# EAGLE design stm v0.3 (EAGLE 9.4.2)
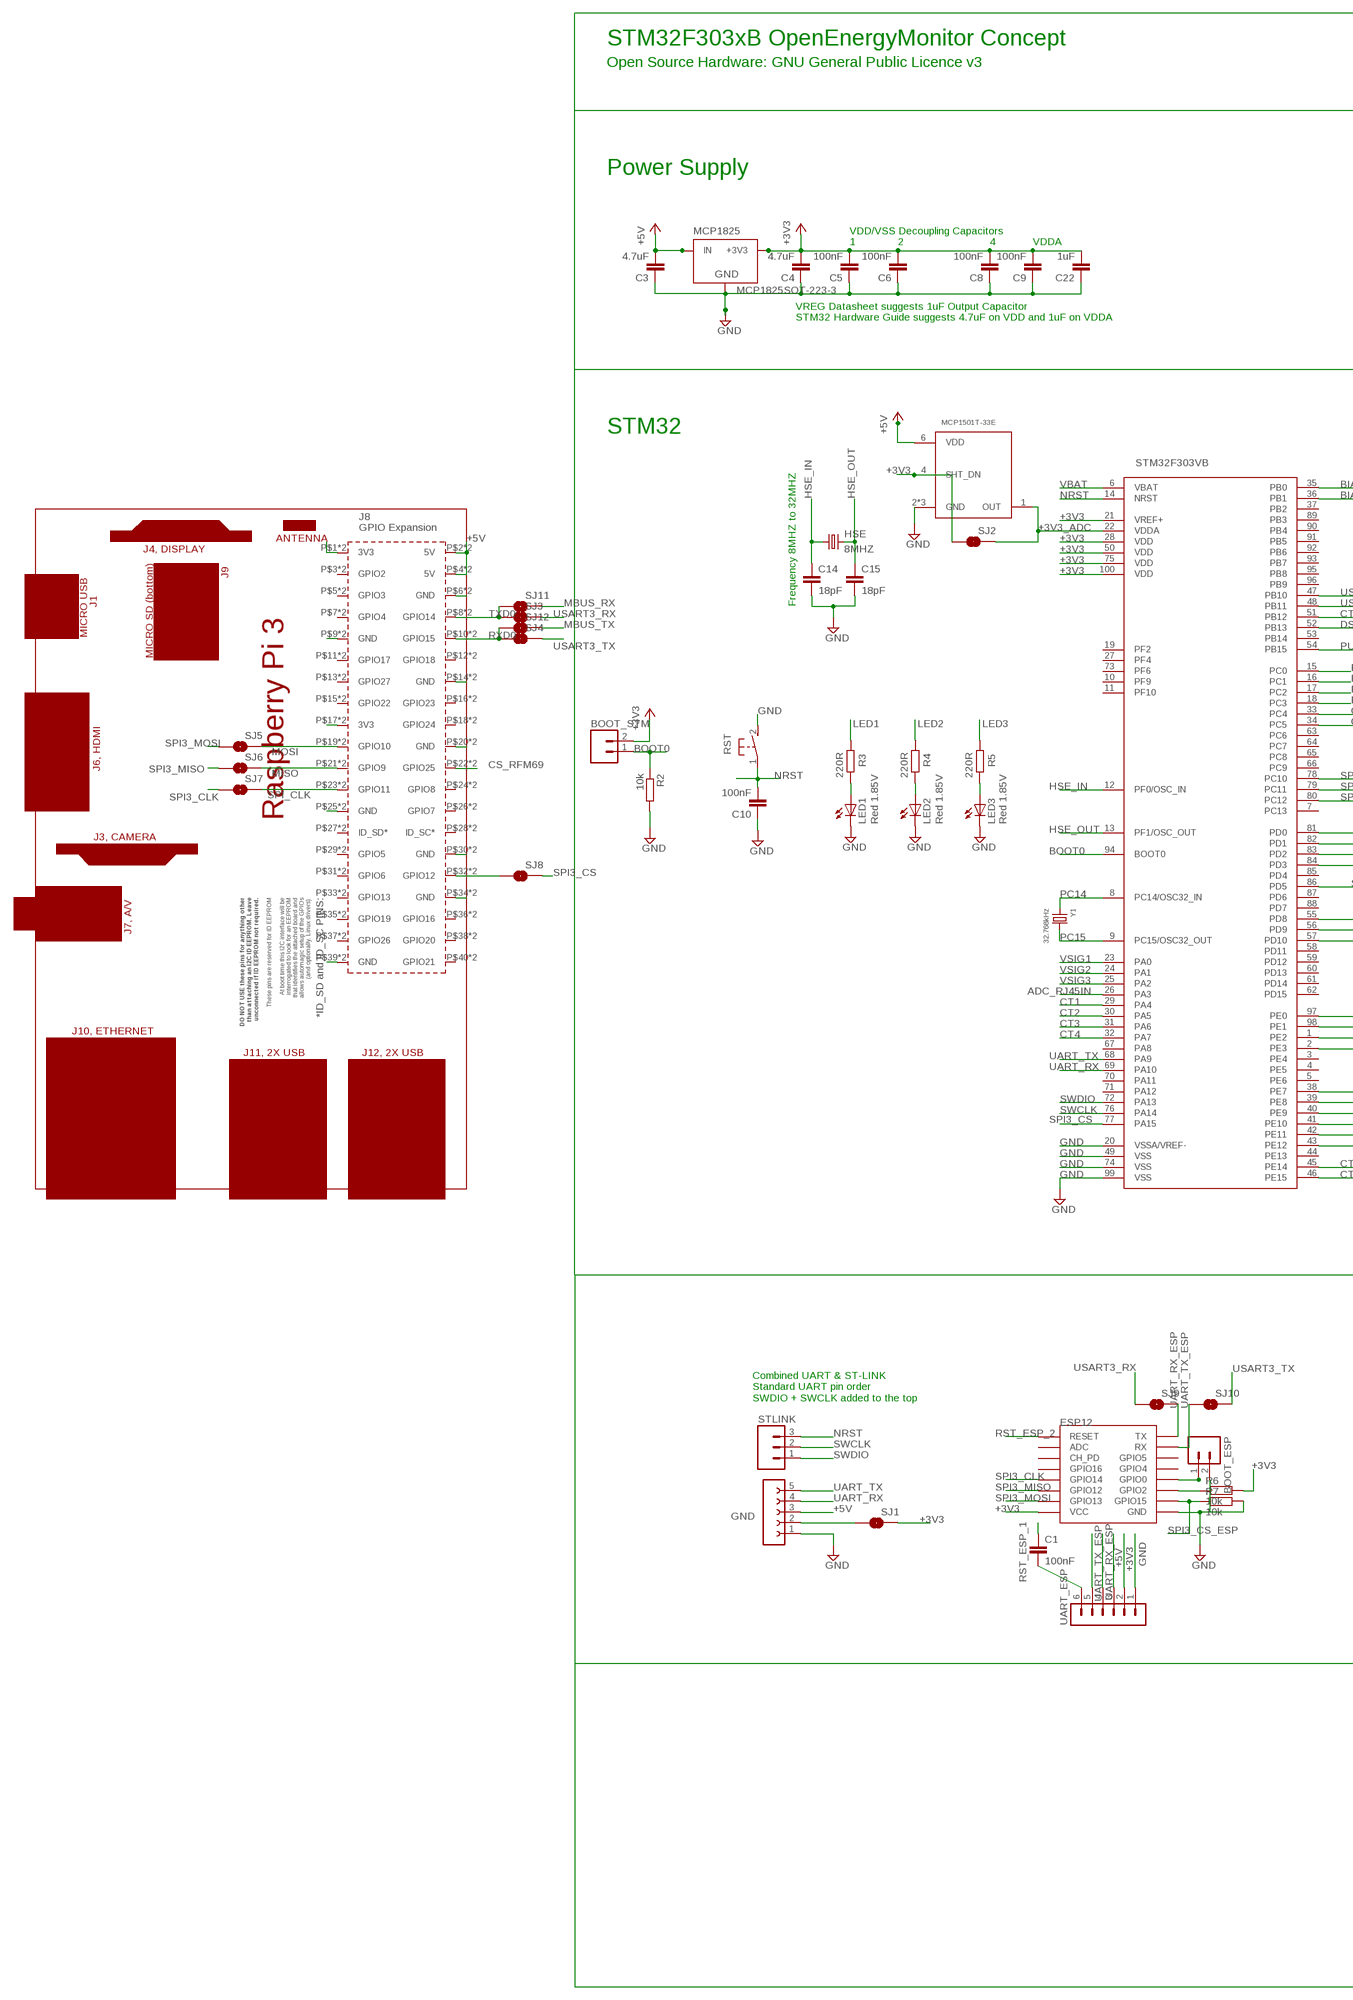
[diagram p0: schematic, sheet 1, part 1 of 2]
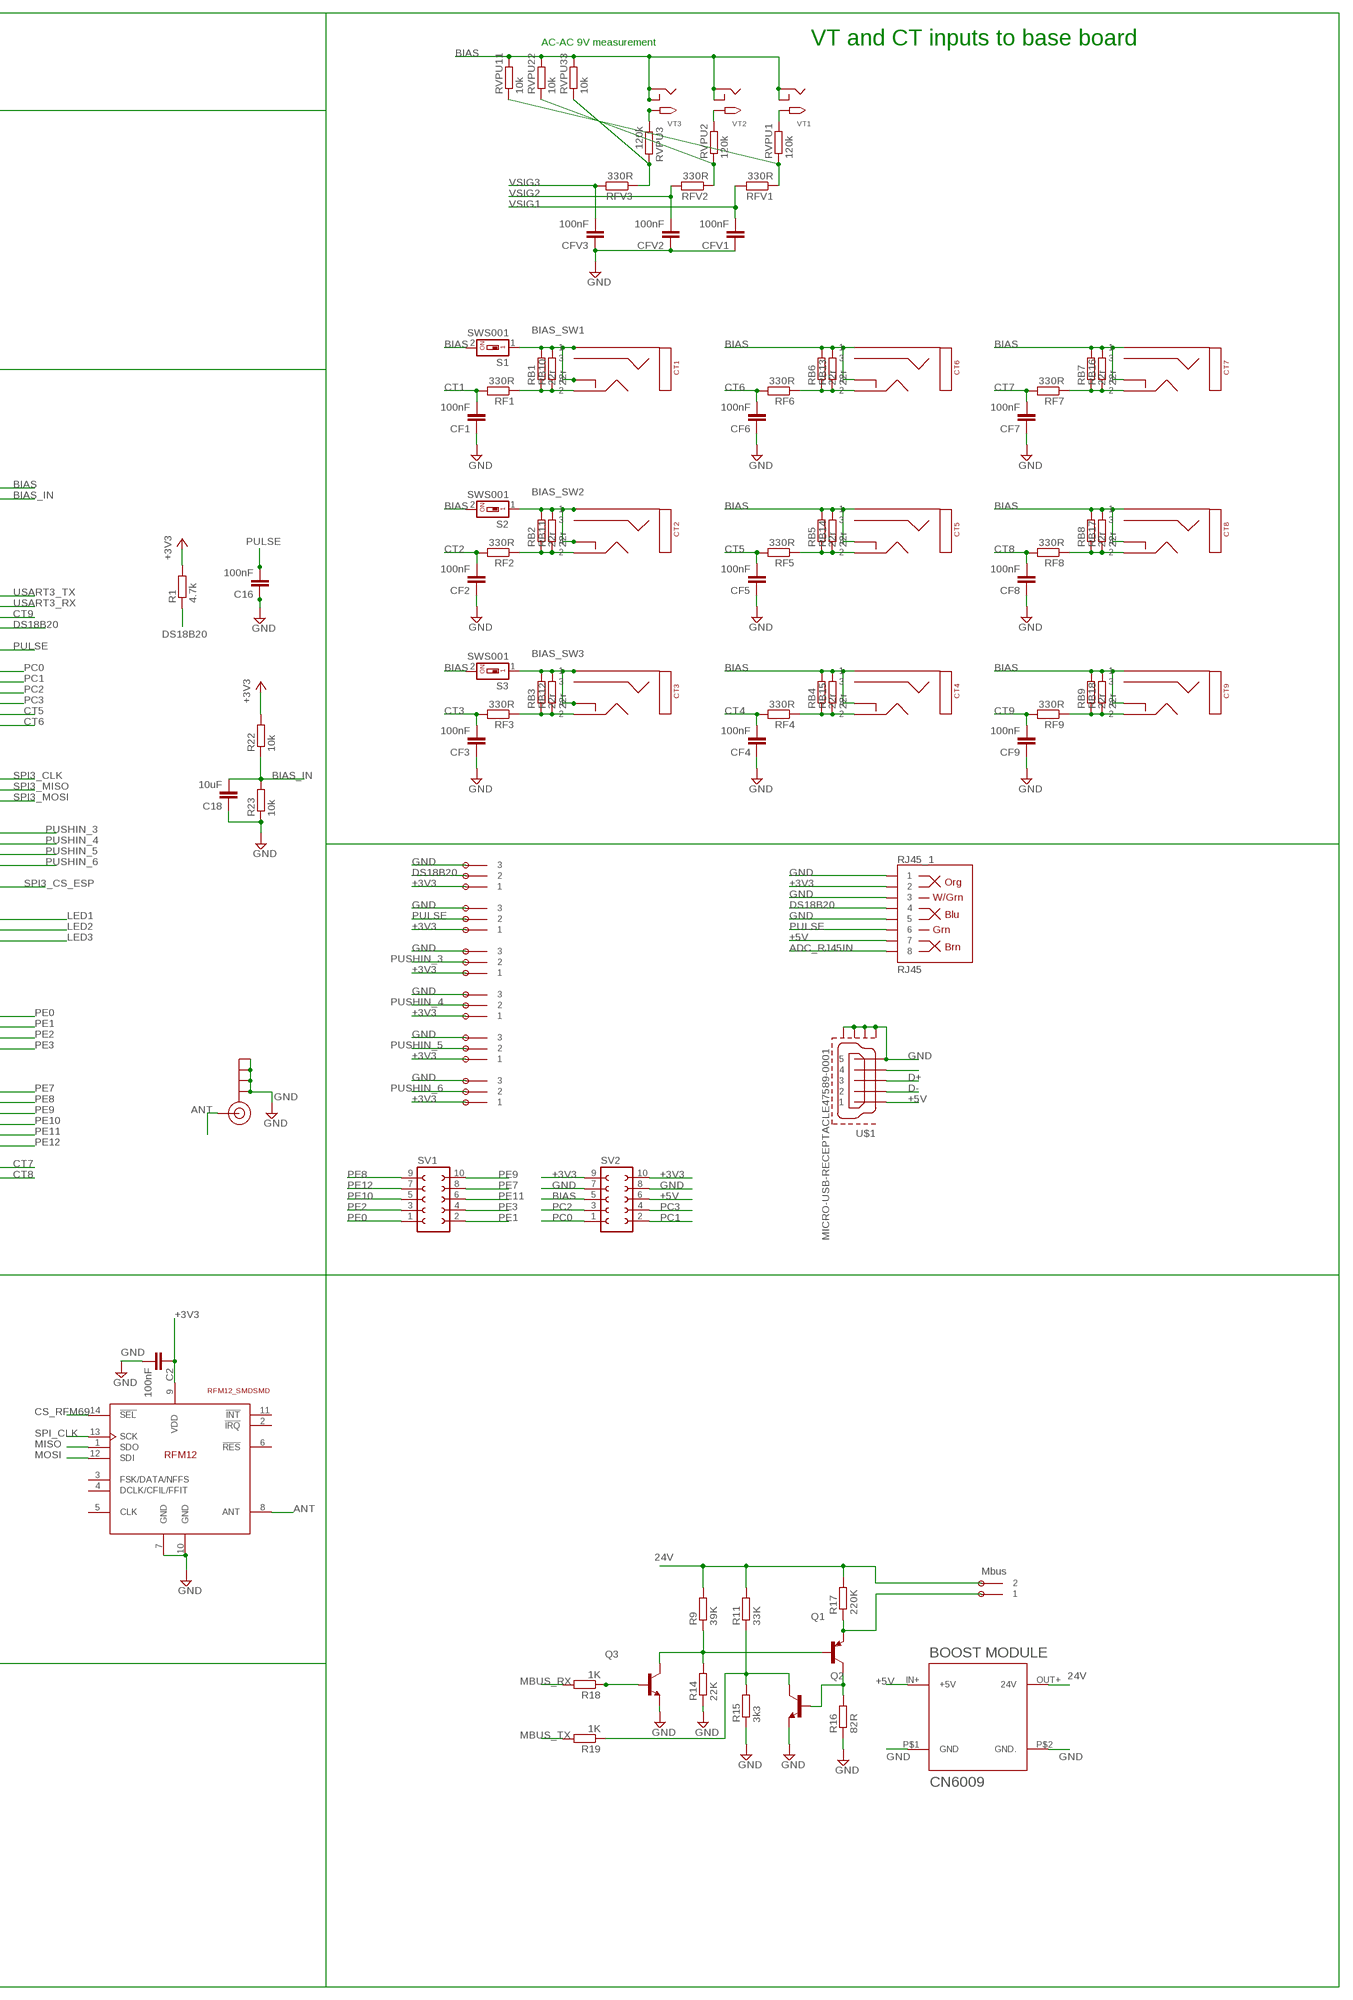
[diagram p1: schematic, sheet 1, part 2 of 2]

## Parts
2POLE_MBUS  OMNIMATE_LSF_2  [OMNIMATE_LSF_2]
3POLE_1  OMNIMATE_LSF_3  [OMNIMATE_LSF_3]
3POLE_2  OMNIMATE_LSF_3  [OMNIMATE_LSF_3]
3POLE_3  OMNIMATE_LSF_3  [OMNIMATE_LSF_3]
3POLE_4  OMNIMATE_LSF_3  [OMNIMATE_LSF_3]
3POLE_5  OMNIMATE_LSF_3  [OMNIMATE_LSF_3]
3POLE_6  OMNIMATE_LSF_3  [OMNIMATE_LSF_3]
BOOT_ESP  M02PTH  [1X02]
BOOT_STM  M02PTH  [1X02]
C1  100nF  C-EUC0603  [C0603]
C2  100nF  C-EUC0603  [C0603]
C3  4.7uF  C-EUC1210  [C1210]
C4  4.7uF  C-EUC1210  [C1210]
C5  100nF  C-EUC0603  [C0603]
C6  100nF  C-EUC0603  [C0603]
C8  100nF  C-EUC0603  [C0603]
C9  100nF  C-EUC0603  [C0603]
C10  100nF  C-EUC0603  [C0603]
C14  18pF  C-EUC0603  [C0603]
C15  18pF  C-EUC0603  [C0603]
C16  100nF  C-EUC0603  [C0603]
C18  10uF  C-EUC0603  [C0603]
C22  1uF  C-EUC1210  [C1210]
CF1  100nF  C-EUC0603  [C0603]
CF2  100nF  C-EUC0603  [C0603]
CF3  100nF  C-EUC0603  [C0603]
CF4  100nF  C-EUC0603  [C0603]
CF5  100nF  C-EUC0603  [C0603]
CF6  100nF  C-EUC0603  [C0603]
CF7  100nF  C-EUC0603  [C0603]
CF8  100nF  C-EUC0603  [C0603]
CF9  100nF  C-EUC0603  [C0603]
CFV1  100nF  C-EUC0603  [C0603]
CFV2  100nF  C-EUC0603  [C0603]
CFV3  100nF  C-EUC0603  [C0603]
CT1  STEREO_SMD  [STEREO_SMT]
CT2  STEREO_SMD  [STEREO_SMT]
CT3  STEREO_SMD  [STEREO_SMT]
CT4  STEREO_SMD  [STEREO_SMT]
CT5  STEREO_SMD  [STEREO_SMT]
CT6  STEREO_SMD  [STEREO_SMT]
CT7  STEREO_SMD  [STEREO_SMT]
CT8  STEREO_SMD  [STEREO_SMT]
CT9  STEREO_SMD  [STEREO_SMT]
ESP12  ESP12SMD  [ESP12-SMD]
GND  UART  FE05-1  [FE05-1]
HSE  8MHZ  CRYSTALCTS406  [CTS406]
J$1  SMA_EDGE  [SMA-EDGE]
LED1  Red 1.85V  LEDCHIP-LED0805  [CHIP-LED0805]
LED2  Red 1.85V  LEDCHIP-LED0805  [CHIP-LED0805]
LED3  Red 1.85V  LEDCHIP-LED0805  [CHIP-LED0805]
MCP1825  MCP1825SOT-223-3  [SOT-223]
PCB2  RPI3YA  [RPI3MIRROR2]
Q1  MMBT3906  [SOT23]
Q2  MMBT3904  [SOT23]
Q3  MMBT3904  [SOT23]
R1  4.7k  R-EU_R0603  [R0603]
R2  10k  R-EU_R0603  [R0603]
R3  220R  R-EU_R0603  [R0603]
R4  220R  R-EU_R0603  [R0603]
R5  220R  R-EU_R0603  [R0603]
R6  10k  R-EU_R0603  [R0603]
R7  10k  R-EU_R0603  [R0603]
R9  39K  R-EU_R0603  [R0603]
R11  33K  R-EU_R0603  [R0603]
R14  22K  R-EU_R0603  [R0603]
R15  3k3  R-EU_R0603  [R0603]
R16  82R  R-EU_R0603  [R0603]
R17  220K  R-EU_R0603  [R0603]
R18  1K  R-EU_R0603  [R0603]
R19  1K  R-EU_R0603  [R0603]
R22  10k  R-EU_R0603  [R0603]
R23  10k  R-EU_R0603  [R0603]
RB1  22r  R-EU_R0603  [R0603]
RB2  22r  R-EU_R0603  [R0603]
RB3  22r  R-EU_R0603  [R0603]
RB4  22r  R-EU_R0603  [R0603]
RB5  22r  R-EU_R0603  [R0603]
RB6  22r  R-EU_R0603  [R0603]
RB7  22r  R-EU_R0603  [R0603]
RB8  22r  R-EU_R0603  [R0603]
RB9  22r  R-EU_R0603  [R0603]
RB10  22r  R-EU_0207/7  [0207/7]
RB11  22r  R-EU_0207/7  [0207/7]
RB12  22r  R-EU_0207/7  [0207/7]
RB13  22r  R-EU_0207/7  [0207/7]
RB14  22r  R-EU_0207/7  [0207/7]
RB15  22r  R-EU_0207/7  [0207/7]
RB16  22r  R-EU_0207/7  [0207/7]
RB17  22r  R-EU_0207/7  [0207/7]
RB18  22r  R-EU_0207/7  [0207/7]
RF1  330R  R-EU_R0603  [R0603]
RF2  330R  R-EU_R0603  [R0603]
RF3  330R  R-EU_R0603  [R0603]
RF4  330R  R-EU_R0603  [R0603]
RF5  330R  R-EU_R0603  [R0603]
RF6  330R  R-EU_R0603  [R0603]
RF7  330R  R-EU_R0603  [R0603]
RF8  330R  R-EU_R0603  [R0603]
RF9  330R  R-EU_R0603  [R0603]
RFM69HCW  RFM12_SMDSMD  [RFM12]
RFV1  330R  R-EU_R0603  [R0603]
RFV2  330R  R-EU_R0603  [R0603]
RFV3  330R  R-EU_R0603  [R0603]
RJ45_1  RJ45  RJ45-8  [RJ45-8]
RST  31-XX  [B3F-31XX]
RVPU1  120k  R-EU_R0603  [R0603]
RVPU2  120k  R-EU_R0603  [R0603]
RVPU3  120k  R-EU_R0603  [R0603]
RVPU11  10k  R-EU_R0603  [R0603]
RVPU22  10k  R-EU_R0603  [R0603]
RVPU33  10k  R-EU_R0603  [R0603]
S1  SWS001  [SMS-001]
S2  SWS001  [SMS-001]
S3  SWS001  [SMS-001]
SJ1  SOLDERJUMPERNO  [SJ_2S-NO]
SJ2  SOLDERJUMPERNO  [SJ_2S-NO]
SJ3  SOLDERJUMPERNO  [SJ_2S-NO]
SJ4  SOLDERJUMPERNO  [SJ_2S-NO]
SJ5  SOLDERJUMPERNO  [SJ_2S-NO]
SJ6  SOLDERJUMPERNO  [SJ_2S-NO]
SJ7  SOLDERJUMPERNO  [SJ_2S-NO]
SJ8  SOLDERJUMPERNO  [SJ_2S-NO]
SJ9  SOLDERJUMPERNO  [SJ_2S-NO]
SJ10  SOLDERJUMPERNO  [SJ_2S-NO]
SJ11  SOLDERJUMPERNO  [SJ_2S-NO]
SJ12  SOLDERJUMPERNO  [SJ_2S-NO]
STLINK  M03PTH  [1X03]
STM32F303VB  STM32F303XB  [TQFP100]
SV1  FE05-2  [FE05-2]
SV2  FE05-2  [FE05-2]
U$1  MICRO-USB-RECEPTACLE47589-0001  [47589-0001]
U$2  BOOST_MODULE  [BOOST]
U$8  MCP1501T-33E  [SOT95P280X145-6N]
UART_ESP  MA06-1  [MA06-1]
VT1  2.1MMJACKSMT  [DCJACK_2MM_SMT]
VT2  2.1MMJACKSMT  [DCJACK_2MM_SMT]
VT3  2.1MMJACKSMT  [DCJACK_2MM_SMT]
Y1  32.768kHz  CRYSTAL8X3.8SMT  [CRYSTAL_8X3.8]

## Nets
24V: 2POLE_MBUS.P$3 2POLE_MBUS.P$4 R9.2 R11.2 R17.2 U$2.OUT+(24V)
+3V3 [power]: 3POLE_1.P$1 3POLE_1.P$2 3POLE_2.P$1 3POLE_2.P$2 3POLE_3.P$1 3POLE_3.P$2 3POLE_4.P$1 3POLE_4.P$2 3POLE_5.P$1 3POLE_5.P$2 3POLE_6.P$1 3POLE_6.P$2 BOOT_STM.2 C2.1 C4.2 C5.2 C6.2 C8.2 C9.2 C22.2 ESP12.VCC MCP1825.3(+3V3) R1.2 R6.2 R22.2 RFM69HCW.9(VDD) RJ45_1.2 SJ1.2 SJ2.1 STM32F303VB.21(VREF+) STM32F303VB.28(VDD) STM32F303VB.50(VDD) STM32F303VB.75(VDD) STM32F303VB.100(VDD) SV2.9 SV2.10 U$8.4(SHT_DN) UART_ESP.2
+3V3_ADC: SJ2.2 STM32F303VB.22(VDDA) U$8.1(OUT)
+5V [power]: C3.2 GND.3 MCP1825.1(IN) PCB2.P$2(5V) PCB2.P$4(5V) PCB2.P$42(5V) PCB2.P$44(5V) RJ45_1.7 SV2.6 U$1.1 U$2.IN+(+5V) U$8.6(VDD) UART_ESP.3
AC1: RVPU1.2 VT1.PWR2(TIP)
AC2: RVPU2.2 VT2.PWR2(TIP)
AC3: RVPU3.1 VT3.PWR2(TIP)
ADC0: RFV3.1 RVPU3.2 RVPU33.1
ADC_RJ45IN: RJ45_1.8 STM32F303VB.26(PA3)
ANT: J$1.SIG(SIGNAL) RFM69HCW.8(ANT)
BIAS: CT4.P$1 CT4.P$4 CT5.P$1 CT5.P$4 CT6.P$1 CT6.P$4 CT7.P$1 CT7.P$4 CT8.P$1 CT8.P$4 CT9.P$1 CT9.P$4 RB4.2 RB5.2 RB6.2 RB7.2 RB8.2 RB9.2 RB13.2 RB14.2 RB15.2 RB16.2 RB17.2 RB18.2 RVPU11.2 RVPU22.2 RVPU33.2 S1.2 S2.2 S3.2 STM32F303VB.35(PB0) SV2.5 VT1.GND(RING) VT1.GNDBREAK(RING_SW) VT2.GND(RING) VT2.GNDBREAK(RING_SW) VT3.GND(RING) VT3.GNDBREAK(RING_SW)
BIAS_IN: C18.2 R22.1 R23.2 STM32F303VB.36(PB1)
BIAS_SW1: CT1.P$1 CT1.P$4 RB1.2 RB10.2 S1.1
BIAS_SW2: CT2.P$1 CT2.P$4 RB2.2 RB11.2 S2.1
BIAS_SW3: CT3.P$1 CT3.P$4 RB3.2 RB12.2 S3.1
BOOT0: BOOT_STM.1 R2.1 STM32F303VB.94(BOOT0)
CS_RFM69: PCB2.P$22(GPIO25) PCB2.P$62(GPIO25) RFM69HCW.14(!SEL)
CT1: CF1.2 RF1.2 STM32F303VB.29(PA4)
CT2: CF2.2 RF2.2 STM32F303VB.30(PA5)
CT3: CF3.2 RF3.2 STM32F303VB.31(PA6)
CT4: CF4.2 RF4.2 STM32F303VB.32(PA7)
CT5: CF5.2 RF5.2 STM32F303VB.33(PC4)
CT6: CF6.2 RF6.2 STM32F303VB.34(PC5)
CT7: CF7.2 RF7.2 STM32F303VB.45(PE14)
CT8: CF8.2 RF8.2 STM32F303VB.46(PE15)
CT9: CF9.2 RF9.2 STM32F303VB.51(PB12)
D+: U$1.3
D-: U$1.2
DS18B20: 3POLE_1.P$3 3POLE_1.P$4 R1.1 RJ45_1.4 STM32F303VB.52(PB13)
GND [power]: 3POLE_1.P$5 3POLE_1.P$6 3POLE_2.P$5 3POLE_2.P$6 3POLE_3.P$5 3POLE_3.P$6 3POLE_4.P$5 3POLE_4.P$6 3POLE_5.P$5 3POLE_5.P$6 3POLE_6.P$5 3POLE_6.P$6 BOOT_ESP.2 C2.2 C3.1 C4.1 C5.1 C6.1 C8.1 C9.1 C10.1 C14.2 C15.2 C16.1 C18.1 C22.1 CF1.1 CF2.1 CF3.1 CF4.1 CF5.1 CF6.1 CF7.1 CF8.1 CF9.1 CFV1.1 CFV2.1 CFV3.1 ESP12.GND GND.1 J$1.GND@0(GND) J$1.GND@1(GND) J$1.GND@2(GND) J$1.GND@3(GND) LED1.C LED2.C LED3.C MCP1825.2(GND) MCP1825.4(GND) PCB2.P$6(GND) PCB2.P$9(GND) PCB2.P$14(GND) PCB2.P$20(GND) PCB2.P$25(GND) PCB2.P$30(GND) PCB2.P$34(GND) PCB2.P$39(GND) PCB2.P$46(GND) PCB2.P$49(GND) PCB2.P$54(GND) PCB2.P$60(GND) PCB2.P$65(GND) PCB2.P$70(GND) PCB2.P$74(GND) PCB2.P$79(GND) Q2.2(E) Q3.2(E) R2.2 R7.2 R14.1 R15.1 R16.1 R23.1 RFM69HCW.7(GND) RFM69HCW.10(GND) RJ45_1.1 RJ45_1.3 RJ45_1.5 RST.2(S) STM32F303VB.20(VSSA/VREF-) STM32F303VB.49(VSS) STM32F303VB.74(VSS) STM32F303VB.99(VSS) SV2.7 SV2.8 U$1.5 U$1.CASING1(GND1) U$1.CASING2(GND2) U$1.CASING3(GND3) U$1.CASING4(GND4) U$2.P$1(GND) U$2.P$2(GND.) U$8.2(GND) U$8.3(GND) U$8.5(GND) UART_ESP.1
HSE_IN: C14.1 HSE.1 STM32F303VB.12(PF0/OSC_IN)
HSE_OUT: C15.1 HSE.3 STM32F303VB.13(PF1/OSC_OUT)
LED1: R3.2 STM32F303VB.55(PD8)
LED2: R4.2 STM32F303VB.56(PD9)
LED3: R5.2 STM32F303VB.57(PD10)
MBUS_RX: R18.2 SJ11.2
MBUS_TX: R19.2 SJ12.2
MISO: PCB2.P$21(GPIO9) PCB2.P$61(GPIO9) RFM69HCW.1(SDO) SJ6.2
MOSI: PCB2.P$19(GPIO10) PCB2.P$59(GPIO10) RFM69HCW.12(SDI) SJ5.2
N$1: GND.2 SJ1.1
N$2: CT1.P$2 RB1.1 RB10.1 RF1.1
N$5: LED2.A R4.1
N$6: LED3.A R5.1
N$7: BOOT_ESP.1 ESP12.GPIO0
N$8: CT2.P$2 RB2.1 RB11.1 RF2.1
N$10: CT3.P$2 RB3.1 RB12.1 RF3.1
N$11: ESP12.GPIO2 R6.1
N$12: U$1.4
N$16: PCB2.P$32(GPIO12) PCB2.P$72(GPIO12) SJ8.1
N$22: PCB2.P$1(3V3) PCB2.P$41(3V3)
N$24: PCB2.P$17(3V3) PCB2.P$57(3V3)
N$29: 2POLE_MBUS.P$1 2POLE_MBUS.P$2 Q1.2(E) R17.1
N$30: Q1.3(C) Q2.1(B) R16.2
N$31: Q1.1(B) Q3.3(C) R9.1 R14.2
N$32: Q2.3(C) R11.1 R15.2 R19.1
N$33: Q3.1(B) R18.1
N$34: RFV2.1 RVPU2.1 RVPU22.1
N$37: RFV1.1 RVPU1.1 RVPU11.1
N$38: CT4.P$2 RB4.1 RB15.1 RF4.1
N$39: CT5.P$2 RB5.1 RB14.1 RF5.1
N$40: CT6.P$2 RB6.1 RB13.1 RF6.1
N$41: LED1.A R3.1
N$42: CT7.P$2 RB7.1 RB16.1 RF7.1
N$43: CT8.P$2 RB8.1 RB17.1 RF8.1
N$44: CT9.P$2 RB9.1 RB18.1 RF9.1
NRST: C10.2 RST.1(P) STLINK.3 STM32F303VB.14(NRST)
PC0: STM32F303VB.15(PC0) SV2.1
PC1: STM32F303VB.16(PC1) SV2.2
PC2: STM32F303VB.17(PC2) SV2.3
PC3: STM32F303VB.18(PC3) SV2.4
PC14: STM32F303VB.8(PC14/OSC32_IN) Y1.P$1
PC15: STM32F303VB.9(PC15/OSC32_OUT) Y1.P$4
PE0: STM32F303VB.97(PE0) SV1.1
PE1: STM32F303VB.98(PE1) SV1.2
PE2: STM32F303VB.1(PE2) SV1.3
PE3: STM32F303VB.2(PE3) SV1.4
PE7: STM32F303VB.38(PE7) SV1.8
PE8: STM32F303VB.39(PE8) SV1.9
PE9: STM32F303VB.40(PE9) SV1.10
PE10: STM32F303VB.41(PE10) SV1.5
PE11: STM32F303VB.42(PE11) SV1.6
PE12: STM32F303VB.43(PE12) SV1.7
PULSE: 3POLE_2.P$3 3POLE_2.P$4 C16.2 RJ45_1.6 STM32F303VB.54(PB15)
PUSHIN_3: 3POLE_3.P$3 3POLE_3.P$4 STM32F303VB.81(PD0)
PUSHIN_4: 3POLE_4.P$3 3POLE_4.P$4 STM32F303VB.82(PD1)
PUSHIN_5: 3POLE_5.P$3 3POLE_5.P$4 STM32F303VB.83(PD2)
PUSHIN_6: 3POLE_6.P$3 3POLE_6.P$4 STM32F303VB.84(PD3)
RST_ESP_1: C1.2 UART_ESP.6
RST_ESP_2: C1.1 ESP12.RESET
RXD0: PCB2.P$10(GPIO15) PCB2.P$50(GPIO15) SJ4.1 SJ12.1
SPI3_CLK: ESP12.GPIO14 SJ7.1 STM32F303VB.78(PC10)
SPI3_CS: SJ8.2 STM32F303VB.77(PA15)
SPI3_CS_ESP: ESP12.GPIO15 R7.1 STM32F303VB.86(PD5)
SPI3_MISO: ESP12.GPIO12 SJ6.1 STM32F303VB.79(PC11)
SPI3_MOSI: ESP12.GPIO13 SJ5.1 STM32F303VB.80(PC12)
SPI_CLK: PCB2.P$23(GPIO11) PCB2.P$63(GPIO11) RFM69HCW.13(SCK) SJ7.2
SWCLK: STLINK.2 STM32F303VB.76(PA14)
SWDIO: STLINK.1 STM32F303VB.72(PA13)
TXD0: PCB2.P$8(GPIO14) PCB2.P$48(GPIO14) SJ3.1 SJ11.1
UART_RX: GND.4 STM32F303VB.69(PA10)
UART_RX_ESP: ESP12.TXD0(TX) SJ9.2 UART_ESP.4
UART_TX: GND.5 STM32F303VB.68(PA9)
UART_TX_ESP: ESP12.RXD0(RX) SJ10.1 UART_ESP.5
USART3_RX: SJ3.2 SJ9.1 STM32F303VB.48(PB11)
USART3_TX: SJ4.2 SJ10.2 STM32F303VB.47(PB10)
VBAT: STM32F303VB.6(VBAT)
VSIG1: CFV1.2 RFV1.2 STM32F303VB.23(PA0)
VSIG2: CFV2.2 RFV2.2 STM32F303VB.24(PA1)
VSIG3: CFV3.2 RFV3.2 STM32F303VB.25(PA2)
Unconnected: CT1.P$3 CT2.P$3 CT3.P$3 CT4.P$3 CT5.P$3 CT6.P$3 CT7.P$3 CT8.P$3 CT9.P$3 ESP12.ADC ESP12.CH_PD ESP12.GPIO4 ESP12.GPIO5 ESP12.GPIO16 PCB2.P$3(GPIO2) PCB2.P$5(GPIO3) PCB2.P$7(GPIO4) PCB2.P$11(GPIO17) PCB2.P$12(GPIO18) PCB2.P$13(GPIO27) PCB2.P$15(GPIO22) PCB2.P$16(GPIO23) PCB2.P$18(GPIO24) PCB2.P$24(GPIO8) PCB2.P$26(GPIO7) PCB2.P$27(ID_SD*) PCB2.P$28(ID_SC*) PCB2.P$29(GPIO5) PCB2.P$31(GPIO6) PCB2.P$33(GPIO13) PCB2.P$35(GPIO19) PCB2.P$36(GPIO16) PCB2.P$37(GPIO26) PCB2.P$38(GPIO20) PCB2.P$40(GPIO21) PCB2.P$43(GPIO2) PCB2.P$45(GPIO3) PCB2.P$47(GPIO4) PCB2.P$51(GPIO17) PCB2.P$52(GPIO18) PCB2.P$53(GPIO27) PCB2.P$55(GPIO22) PCB2.P$56(GPIO23) PCB2.P$58(GPIO24) PCB2.P$64(GPIO8) PCB2.P$66(GPIO7) PCB2.P$67(ID_SD*) PCB2.P$68(ID_SC*) PCB2.P$69(GPIO5) PCB2.P$71(GPIO6) PCB2.P$73(GPIO13) PCB2.P$75(GPIO19) PCB2.P$76(GPIO16) PCB2.P$77(GPIO26) PCB2.P$78(GPIO20) PCB2.P$80(GPIO21) RFM69HCW.2(!IRQ) RFM69HCW.3(FSK/DATA/NFFS) RFM69HCW.4(DCLK/CFIL/FFIT) RFM69HCW.5(CLK) RFM69HCW.6(!RES) RFM69HCW.11(!INT) STM32F303VB.3(PE4) STM32F303VB.4(PE5) STM32F303VB.5(PE6) STM32F303VB.7(PC13) STM32F303VB.10(PF9) STM32F303VB.11(PF10) STM32F303VB.19(PF2) STM32F303VB.27(PF4) STM32F303VB.37(PB2) STM32F303VB.44(PE13) STM32F303VB.53(PB14) STM32F303VB.58(PD11) STM32F303VB.59(PD12) STM32F303VB.60(PD13) STM32F303VB.61(PD14) STM32F303VB.62(PD15) STM32F303VB.63(PC6) STM32F303VB.64(PC7) STM32F303VB.65(PC8) STM32F303VB.66(PC9) STM32F303VB.67(PA8) STM32F303VB.70(PA11) STM32F303VB.71(PA12) STM32F303VB.73(PF6) STM32F303VB.85(PD4) STM32F303VB.87(PD6) STM32F303VB.88(PD7) STM32F303VB.89(PB3) STM32F303VB.90(PB4) STM32F303VB.91(PB5) STM32F303VB.92(PB6) STM32F303VB.93(PB7) STM32F303VB.95(PB8) STM32F303VB.96(PB9)

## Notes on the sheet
- STM32F303xB OpenEnergyMonitor Concept | AC-AC 9V measurement | VT and CT inputs to base board
- Open Source Hardware: GNU General Public Licence v3
- Power Supply
- VDD/VSS Decoupling Capacitors
- 1 | 2 | 4 | VDDA
- VREG Datasheet suggests 1uF Output Capacitor
- STM32 Hardware Guide suggests 4.7uF on VDD and 1uF on VDDA
- STM32
- Frequency 8MHZ to 32MHZ
- Combined UART & ST-LINK
  Standard UART pin order
  SWDIO + SWCLK added to the top
- Mbus

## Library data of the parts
2POLE_MBUS = OMNIMATE_LSF:OMNIMATE_LSF_2
3POLE_1-3POLE_6 = OMNIMATE_LSF:OMNIMATE_LSF_3
BOOT_ESP BOOT_STM = SparkFun:M02: Header 2
C1 C2 C5 C6 C8-C10 C14-C16 C18 CF1-CF9 CFV1-CFV3 = resistor:C-EU: CAPACITOR, European symbol
C3 C4 C22 = rcl:C-EU: CAPACITOR, European symbol; SPICEPREFIX: C
CT1-CT9 = IotaWatt_parts:STEREO_SMD: 3.5mm Stereo Jack SMT
ESP12 = ESP8266 MODULES _ CORRECTED:ESP12: ESP8266 Wifi module 12
GND = con-lsta:FE05-1: FEMALE HEADER; OC_FARNELL: unknown; OC_NEWARK: unknown
HSE = crystal:CRYSTAL: CRYSTAL; OC_FARNELL: unknown; OC_NEWARK: unknown
J$1 = SparkFun-Connectors:SMA_EDGE: SMA Antenna Connector End launch SMA connector. The paste layer has been removed so that the connector can be hand soldered onto the board after reflow.
LED1-LED3 = adafruit:LED: LED
MCP1825 = SteelCaveRobotics-Power:MCP1825: MCP1825 3.3v LDO Linear Regulator
PCB2 = e14_Rpi3_RevA+mirror-pcb copy:RPI3: Device for Raspberry Pi 3 board created by Dave Young for www.element14.com More information and support community is available at https://www.element14.com/community/community/raspberry-pi Device for Raspberry Pi 3 board updated by Gerald Schwarz for www.element14.com On RPI3 addet the layer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
Q1 = Transistor:MMBT3906: TRANS PNP 40V 0.2A SOT-23; CREATED_BY: PCB Layout; DIGIKEY_PART_NUMBER: MMBT3906FSCT-ND; MANUFACTURER: ON Semiconductor; MPN: MMBT3906; PACKAGE: SOT-23
Q2 Q3 = Transistor:MMBT3904: TRANS NPN 40V 0.2A SOT-23; CREATED_BY: PCB Layout; DIGIKEY_PART_NUMBER: MMBT3904FSCT-ND; MANUFACTURER: ON Semiconductor; MPN: MMBT3904; PACKAGE: SOT-23-3
R1 R2 R6 R7 R22 R23 RB1-RB9 RF1-RF9 RFV1-RFV3 RVPU1-RVPU3 RVPU11 RVPU22 RVPU33 = resistor:R-EU_: RESISTOR, European symbol
R3-R5 R9 R11 R14-R19 RB10-RB18 = rcl:R-EU_: RESISTOR, European symbol; SPICEPREFIX: R
RFM69HCW = rfm12b _ rfm69cw:RFM12_SMD: RFM12 is a low costing ISM band transceiver module implemented with unique PLL. It works signal ranges from 315/433/868/915MHZ bands, comply with FCC, ETSI regulation. The SPI interface is used to communicate with microcontroller for parameter setting.
RJ45_1 = SparkFun-Connectors:RJ45-8: RJ45 Jack - 8 pin Simple RJ45, 8-pin connection. Commonly used for Cat5, Cat5e, and Cat6 Ethernet cables. Here is the connector we sell at SparkFun: RJ45 8-Pin Connector (PRT-00643) Datasheet It is used on this SparkFun product: SparkFun RJ45 Breakout (BOB-00716) Note, you may also be interested in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; PROD_ID: CONN-08506; SF_ID: PRT-00643
RST = switch-omron:31-XX: OMRON SWITCH; MPN: B3F-3100; OC_FARNELL: 959704; OC_NEWARK: 36M3582
S1-S3 = smd-special:SWS001: SMD Dip Switch 1 pol.
SJ1-SJ12 = SparkFun:SOLDERJUMPER: Solder Jumper
STLINK = SparkFun:M03: Header 3 Standard 3-pin 0.1" header. Use with straight break away headers (SKU : PRT-00116), right angle break away headers (PRT-00553), swiss pins (PRT-00743), machine pins (PRT-00117), and female headers (PRT-00115). Molex polarized connector foot print use with SKU : PRT-08232 with associated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
STM32F303VB = stm32f303:STM32F303XB
SV1 SV2 = con-lsta-RFM69Pi:FE05-2: FEMALE HEADER; OC_FARNELL: unknown; OC_NEWARK: unknown
U$1 = con-molex-usb:MICRO-USB-RECEPTACLE: MICRO USB RECEPTACLES Micro-USB Receptacles, SMT, Lead-Free from MOLEX. (C) 2014 Tomasz Boleslaw CEDRO, cederom@tlen.pl, http://www.tomek.cedro.info. Version 0.1 (2014-01-17): Initial release. Version 0.2 (2014-02-06): Updated 47589-0001 footprint pins/pads/milling. Following devices are included: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
U$2 = BOOST MODULE CN6009:BOOST_MODULE
U$8 = MCP1501T-33E:MCP1501T-33E
UART_ESP = con-lstb-db:MA06-1: PIN HEADER; OC_FARNELL: unknown; OC_NEWARK: unknown
VT1-VT3 = adafruit:2.1MMJACK: 2.1mm x 5.5mm THM DC jack with internal switch. Digikey part #PJ-102A, 4UCON part #05537 2.1mm x 5.5mm SMT DC jack with internal switch. Digikey part #PJ-002A-SMT, 4UCON part #03267 By microbuilder.eu & adafruit.com
Y1 = microbuilder:CRYSTAL: Crystals

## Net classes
0 default: width 0.254 mm, drill 0.35 mm, clearance 0.152 mm
1 power: width 0.279 mm, drill 0.35 mm, clearance 0.178 mm
2 gnd: width 0.254 mm, drill 0.35 mm, clearance 0.152 mm

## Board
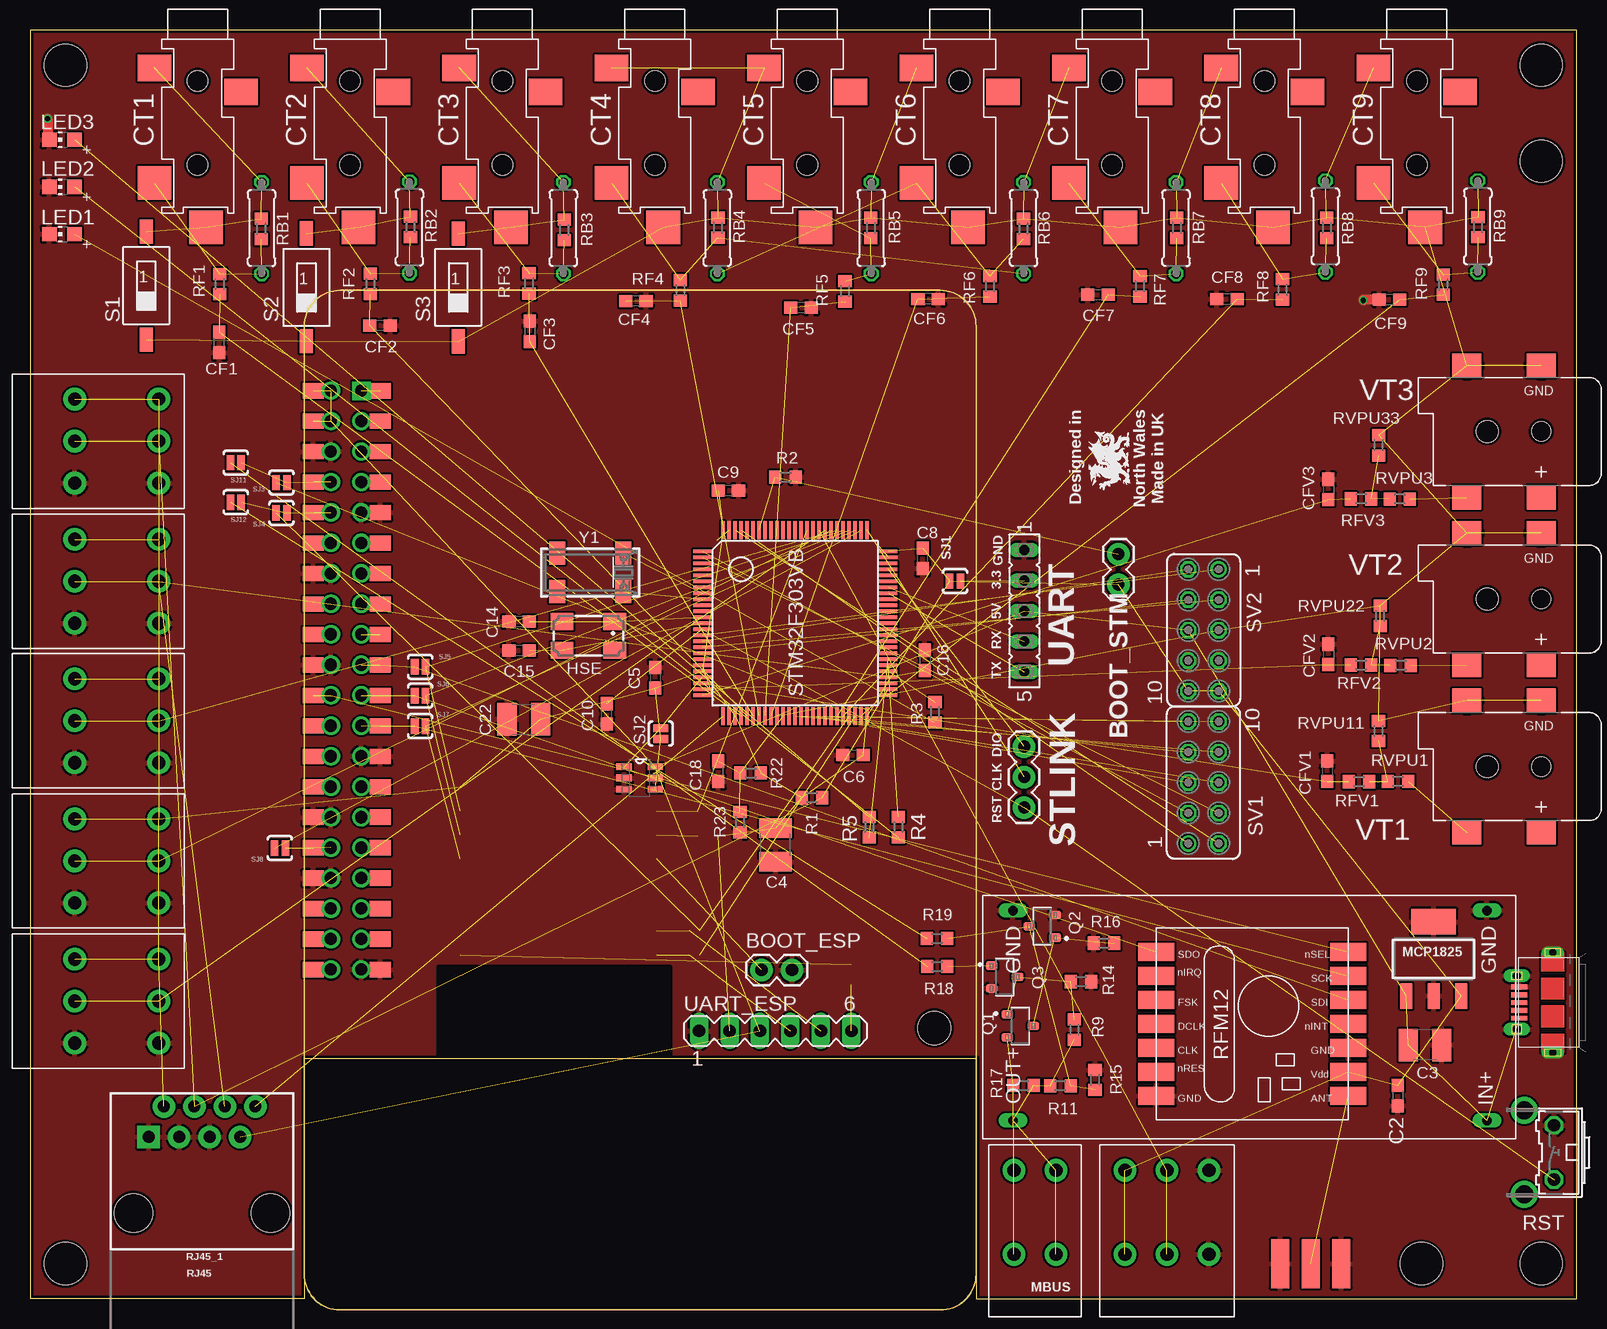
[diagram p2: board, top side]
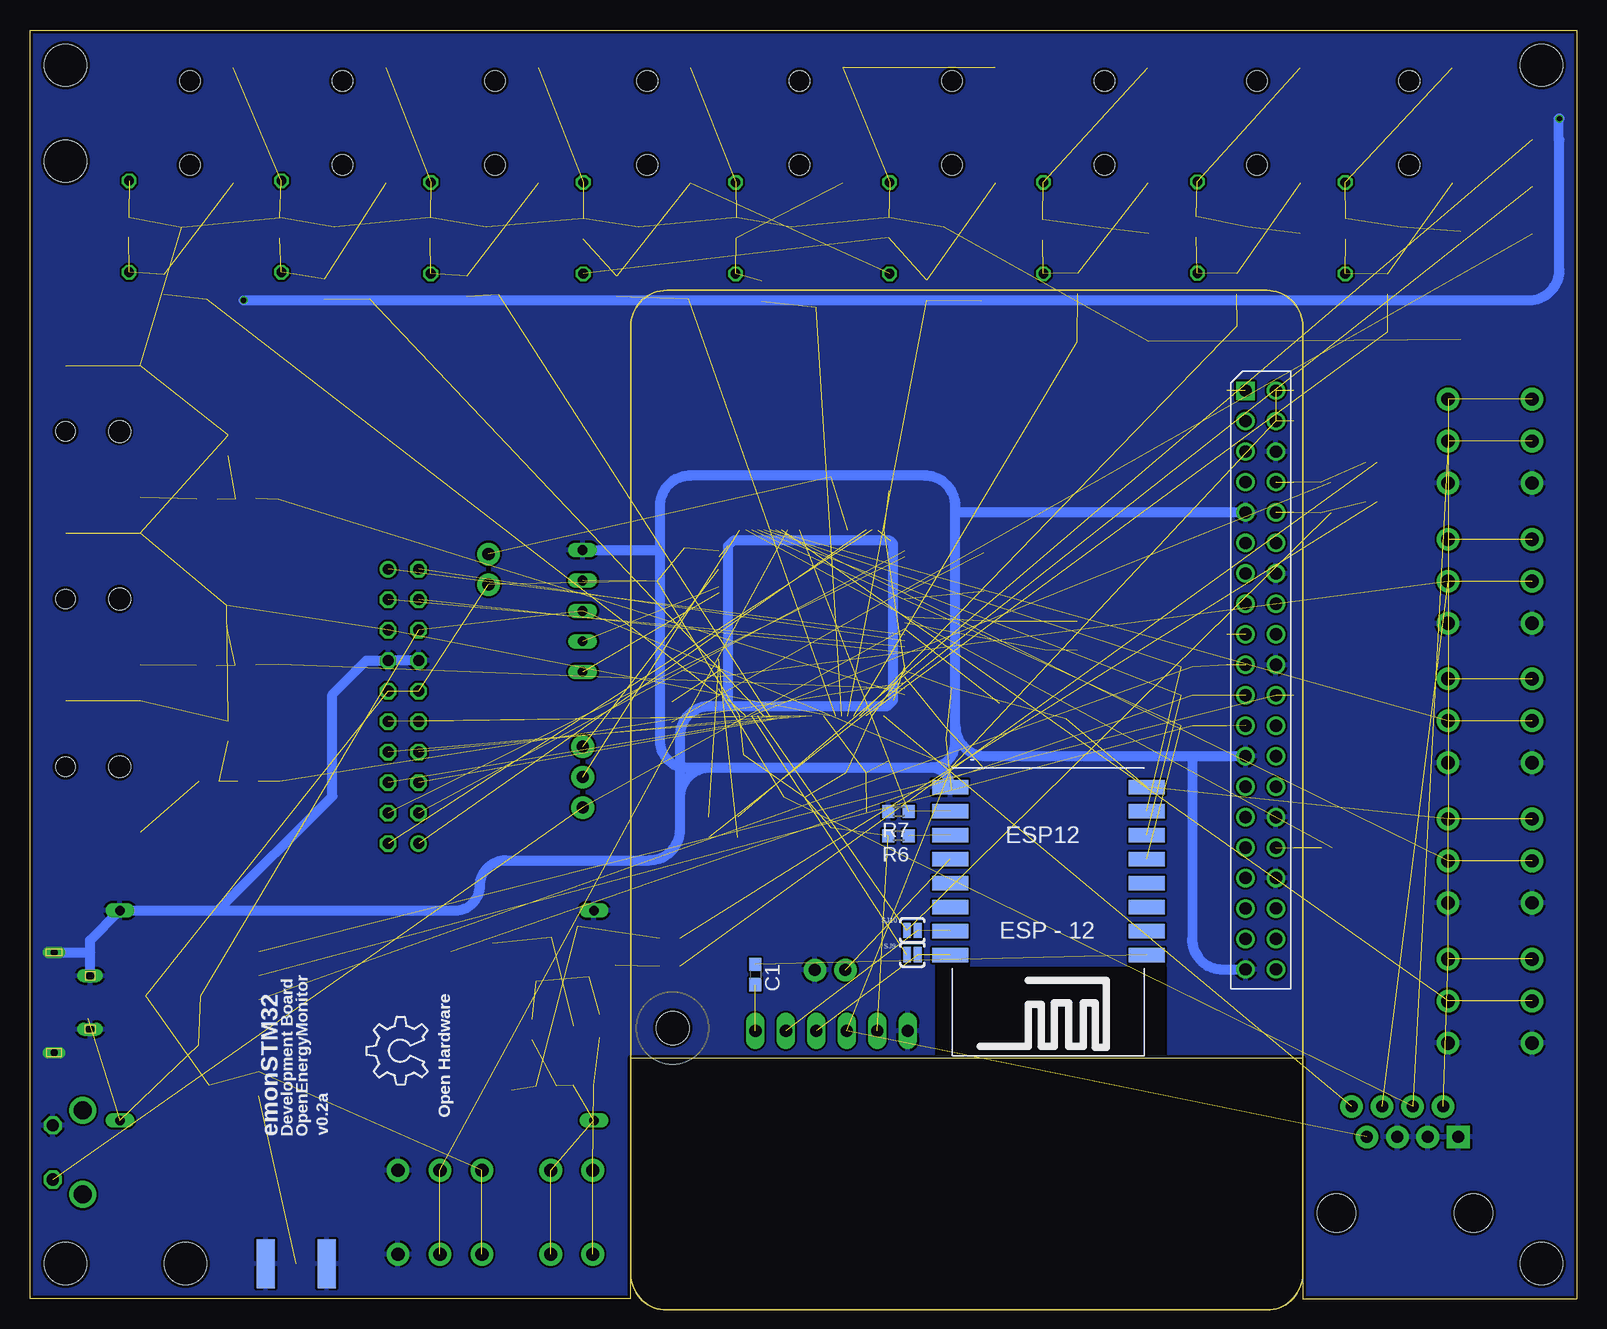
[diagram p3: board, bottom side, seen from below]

Size 128.91 x 105.79 mm. Coordinates in mm from the lower left corner, seen from the top.
Outline: 128.91,105.79 0,105.79 0,0 22.86,0 22.86,20.07 78.87,20.07 78.87,0 128.91,0 128.91,105.79
Copper layers (1*16): Top 0.035mm / dielectric 1.53mm / Bottom 0.035mm
Design rules "jlcpcb *": minimum track width 6mil, minimum drill 0.45mm, track to track 6mil, track to pad 6mil, pad to pad 6mil, via to via 6mil, smd to smd 0mil, copper to edge 10mil, drill to drill 10mil, minimum pad ring 3mil, minimum via ring 3mil, stop-mask expansion 2mil, vias tented up to drill 25mil, thermal gap 8mil
Holes 3.5 mm at 125.95,102.85 2.95,102.85 2.95,2.95 125.95,2.95 125.95,94.85 115.95,2.95
tRestrict: area 34,19.3 to 53.3,27.7
bRestrict: area 34.2,19.3 to 53.5,27.7

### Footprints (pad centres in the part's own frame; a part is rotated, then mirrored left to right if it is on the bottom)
OMNIMATE_LSF_2 = drill 1.1 pad 1.9: P$1 -3.5,-3.5; P$2 -3.5,3.5; P$3 0,-3.5; P$4 0,3.5
OMNIMATE_LSF_3 = drill 1.1 pad 1.9: P$1 -3.5,-3.5; P$2 -3.5,3.5; P$3 0,-3.5; P$4 0,3.5; P$5 3.5,-3.5; P$6 3.5,3.5
1X02 = drill 1.016 pad 1.88: 1 0,0; 2 2.54,0
C0603 = smd 1.1 x 1: 1 -0.85,0; 2 0.85,0
C1210 = smd 1.6 x 2.7: 1 -1.4,0; 2 1.4,0
STEREO_SMT = smd 2.8 x 2.2: P$1 -3.6,-2.4; P$3 3.6,-4.4 | smd 2.8 x 2.8: P$2 -3.6,-12; P$4 0.7,-15.7 | hole 1.7: 0,-3.5; 0,-10.5
ESP12-SMD = smd 3 x 1.2: ADC -8.3,3.8; CH_PD -8.3,1.8; GND 8.1,-8.2; GPIO0 8.1,-2.2; GPIO2 8.1,-4.2; GPIO4 8.1,-0.2; GPIO5 8.1,1.8; GPIO12 -8.3,-4.2; GPIO13 -8.3,-6.2; GPIO14 -8.3,-2.2; GPIO15 8.1,-6.2; GPIO16 -8.3,-0.2; RESET -8.3,5.8; RXD0 8.1,3.8; TXD0 8.1,5.8; VCC -8.3,-8.2
FE05-1 = drill 0.813 long: 1 -5.08,0; 2 -2.54,0; 3 0,0; 4 2.54,0; 5 5.08,0
CTS406 = smd 1.9 x 1.4: 1 -2.2,-1.2; 2 2.2,-1.2; 3 2.2,1.2; 4 -2.2,1.2
SMA-EDGE = smd 1.524 x 4.064: GND@0 0,0; GND@1 5.08,0; SIG 2.54,0 | smd 1.524 x 4.064 bottom: GND@2 0,0; GND@3 5.08,0
CHIP-LED0805 = smd 1.2 x 1.2: A 0,-1.05; C 0,1.05
SOT-223 = smd 1 x 2.1: 1 -2.3,-3.1; 2 0,-3.1; 3 2.3,-3.1 | smd 3.7 x 2.1: 4 0,3.1
RPI3MIRROR2 = drill 1.016 square: P$1 8.37,4.775 | drill 1.016: P$2 8.357,2.233; P$3 10.897,4.773; P$4 10.897,2.233; P$5 13.437,4.773; P$6 13.437,2.233; P$7 15.977,4.773; P$8 15.977,2.233; P$9 18.517,4.773; P$10 18.517,2.233; P$11 21.057,4.773; P$12 21.057,2.233; P$13 23.597,4.773; P$14 23.597,2.233; P$15 26.137,4.773; P$16 26.137,2.233; P$17 28.677,4.773; P$18 28.677,2.233; P$19 31.217,4.773; P$20 31.217,2.233; P$21 33.757,4.773; P$22 33.757,2.233; P$23 36.297,4.773; P$24 36.297,2.233; P$25 38.837,4.773; P$26 38.837,2.233; P$27 41.377,4.773; P$28 41.377,2.233; P$29 43.917,4.773; P$30 43.917,2.233; P$31 46.457,4.773; P$32 46.457,2.233; P$33 48.997,4.773; P$34 48.997,2.233; P$35 51.537,4.773; P$36 51.537,2.233; P$37 54.077,4.773; P$38 54.077,2.233; P$39 56.617,4.773; P$40 56.617,2.233 | smd 1.27 x 1.778: P$41 8.371,6.351; P$42 8.371,0.763; P$43 10.911,6.351; P$44 10.911,0.763; P$45 13.451,6.351; P$46 13.451,0.763; P$47 15.991,6.351; P$48 15.991,0.763; P$49 18.531,6.351; P$50 18.531,0.763; P$51 21.071,6.351; P$52 21.071,0.763; P$53 23.611,6.351; P$54 23.611,0.763; P$55 26.151,6.351; P$56 26.151,0.763; P$57 28.691,6.351; P$58 28.691,0.763; P$59 31.231,6.351; P$60 31.231,0.763; P$61 33.771,6.351; P$62 33.771,0.763; P$63 36.311,6.351; P$64 36.311,0.763; P$65 38.851,6.351; P$66 38.851,0.763; P$67 41.391,6.351; P$68 41.391,0.763; P$69 43.931,6.351; P$70 43.931,0.763; P$71 46.471,6.351; P$72 46.471,0.763; P$73 49.011,6.351; P$74 49.011,0.763; P$75 51.551,6.351; P$76 51.551,0.763; P$77 54.091,6.351; P$78 54.091,0.763; P$79 56.631,6.351; P$80 56.631,0.763 | hole 2.75: 61.5,52.505
SOT23 = smd 0.71 x 0.96: 1 -0.95,-1.075; 2 0.95,-1.075; 3 0,1.075
R0603 = smd 1 x 1.1: 1 -0.85,0; 2 0.85,0
0207/7 = drill 0.813 octagon: 1 -3.81,0; 2 3.81,0
RFM12 = smd 1.5 x 3: 1 -5,-10; 2 -3,-10; 3 -1,-10; 4 1,-10; 5 3,-10; 6 5,-10; 7 7,-10; 8 7,6; 9 5,6; 10 3,6; 11 1,6; 12 -1,6; 13 -3,6; 14 -5,6
RJ45-8 = drill 1 pad 1.88 square: 1 -4.445,6.35 | drill 1 pad 1.88: 2 -3.175,8.89; 3 -1.905,6.35; 4 -0.635,8.89; 5 0.635,6.35; 6 1.905,8.89; 7 3.175,6.35; 8 4.445,8.89 | hole 3.2: -5.715,0; 5.715,0
B3F-31XX = drill 1.016 octagon: 1 -2.261,-1.245; 2 2.261,-1.245 | drill 1.499 pad 2.159: 3 -3.505,1.245; 4 3.505,1.245
SMS-001 = smd 1.092 x 2.007: 1 0,-4.496; 2 0,4.496
SJ_2S-NO = smd 0.635 x 1.27: 1 -0.45,0; 2 0.45,0
1X03 = drill 1.016 pad 1.88: 1 0,0; 2 2.54,0; 3 5.08,0
TQFP100 = smd 0.27 x 1.5: 1 -6,-7.75; 2 -5.5,-7.75; 3 -5,-7.75; 4 -4.5,-7.75; 5 -4,-7.75; 6 -3.5,-7.75; 7 -3,-7.75; 8 -2.5,-7.75; 9 -2,-7.75; 10 -1.5,-7.75; 11 -1,-7.75; 12 -0.5,-7.75; 13 0,-7.75; 14 0.5,-7.75; 15 1,-7.75; 16 1.5,-7.75; 17 2,-7.75; 18 2.5,-7.75; 19 3,-7.75; 20 3.5,-7.75; 21 4,-7.75; 22 4.5,-7.75; 23 5,-7.75; 24 5.5,-7.75; 25 6,-7.75; 51 6,7.75; 52 5.5,7.75; 53 5,7.75; 54 4.5,7.75; 55 4,7.75; 56 3.5,7.75; 57 3,7.75; 58 2.5,7.75; 59 2,7.75; 60 1.5,7.75; 61 1,7.75; 62 0.5,7.75; 63 0,7.75; 64 -0.5,7.75; 65 -1,7.75; 66 -1.5,7.75; 67 -2,7.75; 68 -2.5,7.75; 69 -3,7.75; 70 -3.5,7.75; 71 -4,7.75; 72 -4.5,7.75; 73 -5,7.75; 74 -5.5,7.75; 75 -6,7.75 | smd 1.5 x 0.27: 26 7.75,-6; 27 7.75,-5.5; 28 7.75,-5; 29 7.75,-4.5; 30 7.75,-4; 31 7.75,-3.5; 32 7.75,-3; 33 7.75,-2.5; 34 7.75,-2; 35 7.75,-1.5; 36 7.75,-1; 37 7.75,-0.5; 38 7.75,0; 39 7.75,0.5; 40 7.75,1; 41 7.75,1.5; 42 7.75,2; 43 7.75,2.5; 44 7.75,3; 45 7.75,3.5; 46 7.75,4; 47 7.75,4.5; 48 7.75,5; 49 7.75,5.5; 50 7.75,6; 76 -7.75,6; 77 -7.75,5.5; 78 -7.75,5; 79 -7.75,4.5; 80 -7.75,4; 81 -7.75,3.5; 82 -7.75,3; 83 -7.75,2.5; 84 -7.75,2; 85 -7.75,1.5; 86 -7.75,1; 87 -7.75,0.5; 88 -7.75,0; 89 -7.75,-0.5; 90 -7.75,-1; 91 -7.75,-1.5; 92 -7.75,-2; 93 -7.75,-2.5; 94 -7.75,-3; 95 -7.75,-3.5; 96 -7.75,-4; 97 -7.75,-4.5; 98 -7.75,-5; 99 -7.75,-5.5; 100 -7.75,-6
FE05-2 = drill 0.914: 1 -5.08,1.27 | drill 0.914 octagon: 2 -5.08,-1.27; 3 -2.54,1.27; 4 -2.54,-1.27; 5 0,1.27; 6 0,-1.27; 7 2.54,1.27; 8 2.54,-1.27; 9 5.08,1.27; 10 5.08,-1.27
47589-0001 = smd 1.35 x 0.4: 1 2.8,1.3; 2 2.8,0.65; 3 2.8,0; 4 2.8,-0.65; 5 2.8,-1.3 | drill 0.6 pad 0.95 long: CASING1 0,4.175; CASING2 0,-4.175 | drill 0.7 pad 1.1 long: CASING3 3,2.225; CASING4 3,-2.225
BOOST = drill 0.8 long: IN+ 17.5,39.5; OUT+ 17.5,0; P$1 0,0; P$2 0,39.5
SOT95P280X145-6N = smd 1.27 x 0.559: 1 -1.295,0.94; 2 -1.295,0; 3 -1.295,-0.94; 4 1.295,-0.94; 5 1.295,0; 6 1.295,0.94
MA06-1 = drill 1.016 long: 1 -6.35,0; 2 -3.81,0; 3 -1.27,0; 4 1.27,0; 5 3.81,0; 6 6.35,0
DCJACK_2MM_SMT = smd 2.4 x 2: GND 0,-5.5; GNDBREAK 6.2,-5.5; PWR1 0,5.5; PWR2 6.2,5.5 | hole 1.6: 0,0 | hole 1.8: 4.5,0
CRYSTAL_8X3.8 = smd 1.3 x 1.9: P$1 -2.75,-1.6; P$2 2.75,-1.6; P$3 2.75,1.6; P$4 -2.75,1.6

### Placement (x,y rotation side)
2POLE_MBUS  85.5,7.24 0 top
3POLE_1  7.23,71.51 270 top
3POLE_2  7.23,59.83 270 top
3POLE_3  7.23,48.2 270 top
3POLE_4  7.23,36.52 270 top
3POLE_5  7.23,24.83 270 top
3POLE_6  94.74,7.24 0 top
BOOT_ESP  60.96,27.43 0 top
BOOT_STM  90.7,62.09 270 top
C1  68.45,27.05 270 bottom
C2  113.97,16.96 270 top
C3  116.25,21.17 180 top
C4  62.13,37.85 90 top
C5  52.09,51.79 270 top
C6  68.59,45.34 0 top
C8  74.39,61.75 90 top
C9  58.2,67.38 180 top
C10  48.08,48.78 90 top
C14  40.76,56.47 180 top
C15  40.76,54.04 180 top
C16  74.58,53.24 270 top
C18  57.36,43.98 90 top
C22  41.15,48.34 0 top
CF1  15.79,79.74 90 top
CF2  29.17,81.16 180 top
CF3  41.63,80.66 270 top
CF4  50.49,83.19 180 top
CF5  64.25,82.64 180 top
CF6  74.84,83.37 180 top
CF7  89,83.73 0 top
CF8  99.74,83.37 0 top
CF9  113.3,83.33 0 top
CFV1  108.1,44 270 top
CFV2  108.2,53.74 270 top
CFV3  108.2,67.49 270 top
CT1  13.97,105.04 0 top
CT2  26.67,105.04 0 top
CT3  39.37,105.04 0 top
CT4  52.07,105.04 0 top
CT5  64.77,105.04 0 top
CT6  77.47,105.04 0 top
CT7  90.17,105.04 0 top
CT8  102.87,105.04 0 top
CT9  115.57,105.04 0 top
ESP12  44.13,34.47 180 bottom
GND  82.86,57.36 270 top
HSE  46.54,55.29 180 top
J$1  104.18,2.93 0 top
LED1  2.67,88.77 90 top
LED2  2.67,92.71 90 top
LED3  2.67,96.65 90 top
LOGO1  OSHW_LOGO_6MILX0200-NT  [OSHW_6X200_NOTEXT]  95.78,17.86 90 bottom
MCP1825  116.97,28.35 0 top
PCB2  22.84,84.09 270 top
Q1  82.52,22.77 270 top
Q2  84.34,31.07 90 top
Q3  81.21,26.85 270 top
R1  65.18,41.79 180 top
R2  62.97,68.51 0 top
R3  75.41,48.93 90 top
R4  72.36,39.34 90 top
R5  69.95,39.34 270 top
R6  56.52,38.61 180 bottom
R7  56.52,40.64 180 bottom
R9  87.03,22.46 270 top
R11  85.86,17.77 180 top
R14  87.57,26.46 180 top
R15  88.75,18.27 270 top
R16  89.51,29.66 0 top
R17  82.79,17.81 0 top
R18  75.6,27.72 180 top
R19  75.6,30.06 180 top
R22  60.06,43.85 0 top
R23  59.16,39.76 90 top
RB1  19.27,89.22 90 top
RB2  31.71,89.37 90 top
RB3  44.52,89.12 90 top
RB4  57.33,89.31 90 top
RB5  70.07,89.29 90 top
RB6  82.78,89.22 90 top
RB7  95.56,89.3 90 top
RB8  108.07,89.31 90 top
RB9  120.67,89.36 90 top
RB10  19.3,89.28 90 top
RB11  31.62,89.33 90 top
RB12  44.45,89.28 90 top
RB13  57.28,89.28 90 top
RB14  70.1,89.28 90 top
RB15  82.8,89.28 90 top
RB16  95.5,89.28 90 top
RB17  107.95,89.41 90 top
RB18  120.65,89.41 90 top
RF1  15.81,84.6 270 top
RF2  28.36,84.62 270 top
RF3  41.59,84.66 270 top
RF4  54.2,84.09 270 top
RF5  67.92,84.01 270 top
RF6  80,84.41 270 top
RF7  92.5,84.43 270 top
RF8  104.38,84.16 270 top
RF9  117.77,84.56 270 top
RFM69HCW  103.86,23.92 270 top
RFV1  110.75,43.13 180 top
RFV2  110.93,52.85 180 top
RFV3  110.92,66.72 180 top
RJ45_1  14.33,7.17 0 top
RST  125.76,12.21 90 top
RVPU1  114,43.15 0 top
RVPU2  114.22,52.82 0 top
RVPU3  114.15,66.7 180 top
RVPU11  112.38,47.36 90 top
RVPU22  112.52,56.96 90 top
RVPU33  112.39,71.18 90 top
S1  9.69,84.49 180 top
S2  23.04,84.34 180 top
S3  35.69,84.33 180 top
SJ1  77.09,59.85 180 top
SJ2  52.56,47.13 90 top
SJ3  20.95,68.07 180 top
SJ4  20.95,65.53 180 top
SJ5  32.51,52.7 180 top
SJ6  32.51,50.29 180 top
SJ7  32.51,47.75 180 top
SJ8  20.83,37.59 180 top
SJ9  55.37,28.7 0 bottom
SJ10  55.37,30.73 180 bottom
SJ11  17.14,69.72 180 top
SJ12  17.14,66.42 180 top
STLINK  82.84,46.06 270 top
STM32F303VB  63.75,56.34 270 top
SV1  97.79,43.05 90 top
SV2  97.79,55.75 270 top
U$1  126.89,24.71 180 top
U$2  81.92,32.38 270 top
U$8  50.8,43.43 0 top
UART_ESP  62.1,22.35 0 top
VT1  125.94,44.38 180 top
VT2  125.94,58.35 180 top
VT3  125.94,72.32 180 top
Y1  46.69,60.58 180 top

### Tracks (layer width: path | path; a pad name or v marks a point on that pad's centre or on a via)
24V  (5 unrouted)
+3V3  (37 unrouted)
+3V3_ADC  (2 unrouted)
+5V  (12 unrouted)
AC1  (1 unrouted)
AC2  (1 unrouted)
AC3  (1 unrouted)
ADC0  (2 unrouted)
ADC_RJ45IN  (1 unrouted)
ANT  (1 unrouted)
BIAS  (37 unrouted)
BIAS_IN  (3 unrouted)
BIAS_SW1  (4 unrouted)
BIAS_SW2  (4 unrouted)
BIAS_SW3  (4 unrouted)
BOOT0  (2 unrouted)
CS_RFM69  (2 unrouted)
CT1  (2 unrouted)
CT2  (2 unrouted)
CT3  (2 unrouted)
CT4  (2 unrouted)
CT5  (2 unrouted)
CT6  (2 unrouted)
CT7  (2 unrouted)
CT8  (2 unrouted)
CT9  (2 unrouted)
DS18B20  (4 unrouted)
GND  (via drill 0.45)  (4 unrouted)
  Top 0.813: CF9.1 111.18,83.33 arc90 v111.1,83.26 | v1.46,98.4 1.46,96.8 arc90 LED3.C
  Bottom 0.813: U$1.CASING4 123.89,28.86 | 123.89,28.86 123.89,29.91 U$2.P$2 113.24,32.38 | 113.24,32.38 103.72,41.91 103.72,50.39 100.89,53.21 SV2.7 SV2.8 | 70.74,49.97 70.74,62.78 70.3,63.22 57.23,63.22 56.98,62.97 56.98,49.9 57.42,49.46 72.2,49.46 arc-90 74.74,46.92 74.74,41.77 | 113.24,32.38 93.46,32.38 arc-90 91.41,34.44 arc90 89.27,36.58 77.28,36.58 arc-90 74.74,39.12 74.74,41.77 | 74.74,41.77 arc90 72.2,44.31 | ESP12.GND arc-90 53.87,44.31 | 72.2,44.31 53.87,44.31 | 53.87,44.31 arc-90 51.79,46.39 51.79,47.79 | 76.42,62.43 76.42,66.1 arc90 73.88,68.64 54.33,68.64 arc90 51.79,66.1 51.79,65.56 | 76.42,62.43 76.42,46.53 arc-90 74.2,44.31 72.2,44.31 | 51.79,47.79 51.79,65.56 | 51.79,47.79 arc-90 49.25,45.25 32.07,45.25 | 32.07,45.25 PCB2.P$25 | PCB2.P$9 51.77,65.57 arc-90 51.79,65.56 | 32.07,45.25 32.07,30.01 arc-90 29.53,27.47 PCB2.P$39 | v111.1,83.26 3.99,83.26 arc-90 1.45,85.8 1.45,96.57 arc-90 1.53,96.65 1.53,98.33 arc90 v1.46,98.4 | GND.1 76.44,62.44 arc90 76.42,62.43 | U$1.CASING2 123.92,28.89 arc90 123.89,28.86
  pour Top (isolate 0.178): 139.22,-7.21 -8.73,-7.21 -8.73,108.6 139.22,108.6
  pour Bottom: -12.17,110.63 -12.17,-9.99 141.99,-9.99 141.99,110.63
HSE_IN  (2 unrouted)
HSE_OUT  (2 unrouted)
LED1  (1 unrouted)
LED2  (1 unrouted)
LED3  (1 unrouted)
MBUS_RX  (1 unrouted)
MBUS_TX  (1 unrouted)
MISO  (3 unrouted)
MOSI  (3 unrouted)
N$1  (1 unrouted)
N$2  (3 unrouted)
N$5  (1 unrouted)
N$6  (1 unrouted)
N$7  (1 unrouted)
N$8  (3 unrouted)
N$10  (3 unrouted)
N$11  (1 unrouted)
N$16  (2 unrouted)
N$22  (1 unrouted)
N$24  (1 unrouted)
N$29  (3 unrouted)
N$30  (2 unrouted)
N$31  (3 unrouted)
N$32  (3 unrouted)
N$33  (1 unrouted)
N$34  (2 unrouted)
N$37  (2 unrouted)
N$38  (3 unrouted)
N$39  (3 unrouted)
N$40  (3 unrouted)
N$41  (1 unrouted)
N$42  (3 unrouted)
N$43  (3 unrouted)
N$44  (3 unrouted)
NRST  (3 unrouted)
PC0  (1 unrouted)
PC1  (1 unrouted)
PC2  (1 unrouted)
PC3  (1 unrouted)
PC14  (1 unrouted)
PC15  (1 unrouted)
PE0  (1 unrouted)
PE1  (1 unrouted)
PE2  (1 unrouted)
PE3  (1 unrouted)
PE7  (1 unrouted)
PE8  (1 unrouted)
PE9  (1 unrouted)
PE10  (1 unrouted)
PE11  (1 unrouted)
PE12  (1 unrouted)
PULSE  (4 unrouted)
PUSHIN_3  (2 unrouted)
PUSHIN_4  (2 unrouted)
PUSHIN_5  (2 unrouted)
PUSHIN_6  (2 unrouted)
RST_ESP_1  (1 unrouted)
RST_ESP_2  (1 unrouted)
RXD0  (3 unrouted)
SPI3_CLK  (2 unrouted)
SPI3_CS  (1 unrouted)
SPI3_CS_ESP  (2 unrouted)
SPI3_MISO  (2 unrouted)
SPI3_MOSI  (2 unrouted)
SPI_CLK  (3 unrouted)
SWCLK  (1 unrouted)
SWDIO  (1 unrouted)
TXD0  (3 unrouted)
UART_RX  (1 unrouted)
UART_RX_ESP  (2 unrouted)
UART_TX  (1 unrouted)
UART_TX_ESP  (2 unrouted)
USART3_RX  (2 unrouted)
USART3_TX  (2 unrouted)
VSIG1  (2 unrouted)
VSIG2  (2 unrouted)
VSIG3  (2 unrouted)

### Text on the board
tPlace: Designed in | North Wales | Made in UK
bPlace: Open Hardware
tNames: VT3 | SJ1 | VT2 | UART | 3.3 | 5V | RX | TX | DIO | CLK | RST | VT1 | MBUS
bNames: v0.2a | OpenEnergyMonitor | Development Board | emonSTM32
tDocu: 128.905 x / 105.791 y

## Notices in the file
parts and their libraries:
SparkFun-Connectors: Licensing: Creative Commons ShareAlike 4.0 International - https://creativecommons.org/licenses/by-sa/4.0
microbuilder: This work is placed in the public domain, and may be freely used for commercial and non-commercial work with the following conditions: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
